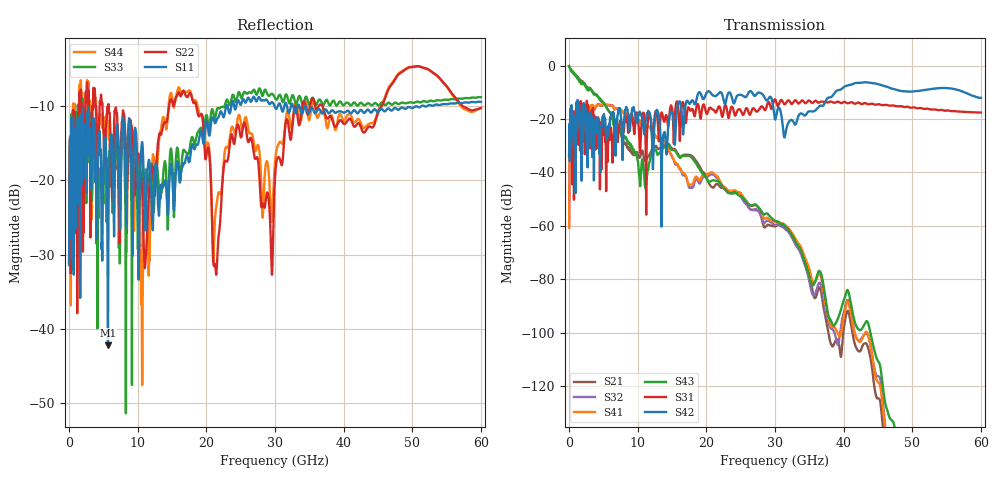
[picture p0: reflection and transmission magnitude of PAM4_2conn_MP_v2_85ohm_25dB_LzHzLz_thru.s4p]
! Info: Touchstone file created by Circ.  Input file=FAB50GbE_2conn_Midplane_Examax_Topo2_v2_85ohm_25dB_LzHzLz.circ
# Hz S RI R 50
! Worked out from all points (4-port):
!   6000 points, 10 MHz to 60 GHz, reference 50 ohm
!   strongest paths, dB at 10 MHz, 15.01 GHz, 30.01 GHz, 45.01 GHz, 60 GHz:
!     S42: -34.0, -17.4, -20.2, -7.0, -12.1
!     S31: -34.0, -16.0, -12.6, -14.5, -17.6
!     S43: -0.2, -31.6, -58.2, -110.6, -169.9
!     S41: -60.7, -34.1, -58.6, -118.5, -172.0
!     S32: -60.7, -34.1, -59.7, -116.4, -167.4
!     S21: -0.2, -31.1, -60.2, -124.7, -167.3
!   lowest |S11| = -42.2 dB at 5.67 GHz (marker M1), VSWR 1.02, Z = 49.5 - j0.553 ohm
!   |S11| at or under -10 dB: start of sweep to 22.89 GHz; 33.56 GHz to 34.36 GHz (803.3 MHz wide, 2.37 % of centre); 34.43 GHz to 51.37 GHz (16.94 GHz wide, 39.5 % of centre)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
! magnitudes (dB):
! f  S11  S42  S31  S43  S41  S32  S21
! 10 MHz  -31.2  -34.0  -34.0  -0.2  -60.7  -60.7  -0.2
! 1 GHz  -13.7  -21.8  -17.1  -4.0  -17.1  -17.0  -3.8
! 5.67 GHz  -42.2  -26.0  -31.0  -16.6  -14.7  -14.9  -16.5
! 17.71 GHz  -16.4  -13.9  -16.9  -34.1  -44.6  -45.7  -33.5
! 21.29 GHz  -12.3  -11.5  -17.4  -43.2  -41.0  -41.5  -44.8
! 35.18 GHz  -10.4  -17.2  -13.5  -80.7  -78.0  -83.0  -80.0
! 60 GHz  -9.5  -12.1  -17.6  -169.9  -172.0  -167.4  -167.3
